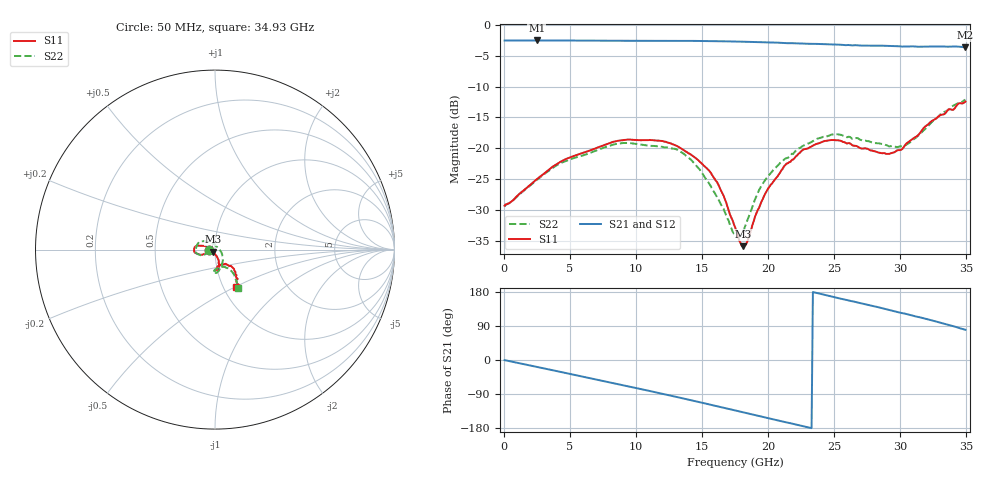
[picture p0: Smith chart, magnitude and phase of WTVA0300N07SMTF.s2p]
! 50 ohm 2-Port S-parameters measured by Modelithics Inc support@modelithics.com  Tampa, FL USA 813-866-6335 (February 2024)
! Smiths Interconnect,  3dB P/N: WTVA0300N07SMTF, Temperature: 50 C
! Board: 10 mil Rogers 4350B, Mounting Pad Dimensions: Length: 15 mils, Width: 25 mils, Gap: 40 mils.
# Hz S RI R 50
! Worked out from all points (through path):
!   352 points, 50 MHz to 34.93 GHz, reference 50 ohm
!   highest |S21| = -2.53 dB at 2.489 GHz (marker M1); lowest = -3.6 dB at 34.93 GHz (marker M2)
!   group delay of S21, straight-line fit = 22.1 ps
!   lowest |S11| = -35.9 dB at 18.11 GHz (marker M3), VSWR 1.03, Z = 48.9 - j1.1 ohm
!   |S11| at or under -10 dB: start of sweep to end of sweep
!   |S22| runs from -34.5 to -12.1 dB; largest |S21 - S12| = 0.0085
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5e7  -0.0341 -7.36e-06  0.7467 -0.00425  0.7458 -0.00419  -0.0335 -0.00134
2.4885e9  -0.0521 -0.0204  0.7104 -0.2329  0.7096 -0.2327  -0.0501 -0.0232
4.18e9  -0.0708 -0.0285  0.6425 -0.3807  0.6417 -0.3804  -0.0673 -0.0322
5.8715e9  -0.0864 -0.0276  0.544 -0.5103  0.5435 -0.5099  -0.0807 -0.0311
8.8565e9  -0.115 -0.0129  0.3097 -0.6755  0.3079 -0.6755  -0.1089 -0.0131
1.1742e10  -0.1145 0.0108  0.0352 -0.7411  0.0337 -0.7404  -0.1003 0.0249
1.36325e10  -0.0934 0.0222  -0.1543 -0.7261  -0.1553 -0.7251  -0.0768 0.046
1.5523e10  -0.0625 0.0205  -0.3368 -0.6582  -0.339 -0.6561  -0.0303 0.0418
1.66175e10  -0.039 0.0136  -0.4317 -0.5963  -0.4326 -0.595  -0.00698 0.0315
1.7513e10  -0.0225 -0.00144  -0.5026 -0.535  -0.5026 -0.5339  0.00824 0.0175
1.78115e10  -0.0168 -0.00554  -0.5247 -0.5108  -0.5239 -0.5104  0.0136 0.0136
1.811e10  -0.0114 -0.0112  -0.5436 -0.4871  -0.543 -0.4866  0.0196 0.00766
1.84085e10  -0.00619 -0.0161  -0.5624 -0.4635  -0.5624 -0.4625  0.0256 0.000506
1.92045e10  0.00399 -0.0311  -0.6081 -0.3953  -0.6072 -0.3953  0.0378 -0.0212
1.9901e10  0.0126 -0.0434  -0.6411 -0.3316  -0.6404 -0.3313  0.0418 -0.0397
2.13935e10  0.0211 -0.0718  -0.6854 -0.1869  -0.6849 -0.186  0.0402 -0.0727
2.33835e10  0.0209 -0.1025  -0.702 0.00825  -0.7013 0.00821  0.0247 -0.1113
2.5274e10  0.0128 -0.1151  -0.6642 0.1956  -0.6635 0.1951  0.00352 -0.1295
2.91545e10  0.0333 -0.0834  -0.4527 0.5003  -0.4475 0.504  0.0151 -0.1022
3.0448e10  0.068 -0.085  -0.3489 0.5695  -0.3433 0.5721  0.0459 -0.0959
3.2836e10  0.1141 -0.1373  -0.1197 0.6584  -0.1165 0.6583  0.1077 -0.1428
3.49255e10  0.1178 -0.2075  0.1172 0.6482  0.1174 0.6471  0.1277 -0.2119
